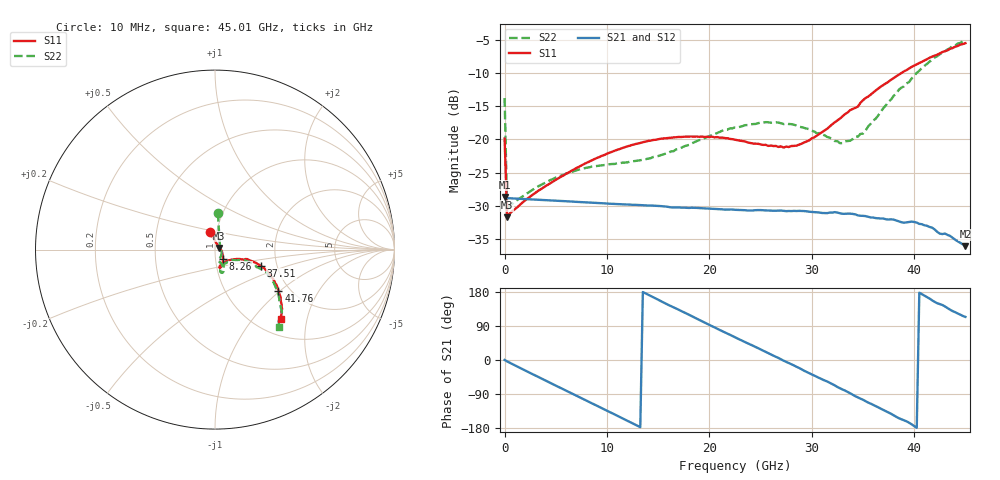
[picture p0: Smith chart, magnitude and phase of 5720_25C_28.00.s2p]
! Device:  ADRF5720
! Description: 0.5dB LSB GaAs MMIC 6-bit Digital Attenuator
! Frequency:  0.000009 -  40 GHz
! Ports:
!	RF1	= Port 1
!	RF2	= Port 2
! Vdd:  3.3 Volt
! Vss:  -3.3 Volt
! Control:  0/3.3 Volt
! State:  28.00 dB attenuation
! Data:  The device was measured using G-S-G Probes on a matrix board.
!  Data was collected using an calibrated 4 port network analyzer.
!  The reference plane for this measurement is at the launchers.
! Note:  Analog Devices supplies this data as a sample of measured data
!  for this product.  Your particular data for this product may vary.
!  Data was taken at 25 degrees C.
!  Analog Devices reserves the right to change this data at anytime.
# GHZ S DB R 45.0
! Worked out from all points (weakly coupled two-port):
!   181 points, 10 MHz to 45.01 GHz, reference 45 ohm
!   highest |S21| = -28.67 dB at 10 MHz (marker M1); lowest = -36.1 dB at 45.01 GHz (marker M2)
!   lowest |S11| = -31.7 dB at 260 MHz (marker M3), VSWR 1.05, Z = 47.2 + j0.883 ohm
!   |S11| at or under -10 dB: start of sweep to 38.75 GHz
!   |S22| runs from -30.6 to -5.1 dB; largest |S21 - S12| = 0.0001
!   S11 on the Smith chart (normalised r, x): 10 MHz: 0.93, +0.18; 8.26 GHz: 1.09, -0.11; 37.51 GHz: 1.65, -0.33; 41.76 GHz: 1.75, -0.97; 45.01 GHz: 1.30, -1.40
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0.01  -19.88 106.9  -28.67 0.1  -28.66 0.1  -13.78 85.6
0.26  -31.71 21.1  -28.85 -3.7  -28.85 -3.7  -30.62 15.6
3.26  -27.78 -17.5  -29.08 -44.3  -29.08 -44.3  -27.10 -35.2
7.76  -23.72 -46.2  -29.47 -104.0  -29.47 -104.0  -24.36 -68.5
8.26  -23.35 -48.5  -29.52 -110.6  -29.51 -110.6  -24.21 -70.0
12.01  -21.04 -62.0  -29.81 -160.4  -29.81 -160.4  -23.45 -74.4
15.26  -19.90 -69.9  -30.05 155.5  -30.05 155.5  -22.37 -68.8
20.26  -19.58 -75.8  -30.46 89.2  -30.46 89.2  -19.35 -63.6
22.76  -20.13 -75.0  -30.63 56.7  -30.63 56.8  -18.18 -66.4
25.51  -20.82 -65.5  -30.70 21.2  -30.70 21.2  -17.40 -71.8
27.26  -21.23 -56.3  -30.76 -1.8  -30.76 -1.8  -17.69 -74.3
30.26  -19.68 -33.4  -30.96 -41.0  -30.96 -41.0  -18.81 -74.5
32.76  -16.87 -21.4  -31.13 -74.6  -31.14 -74.6  -20.57 -60.0
33.76  -15.59 -19.5  -31.19 -87.8  -31.19 -87.8  -20.20 -46.3
34.51  -15.06 -17.3  -31.45 -98.8  -31.45 -98.7  -19.58 -38.7
35.01  -14.10 -17.0  -31.52 -104.9  -31.52 -104.9  -19.13 -33.2
37.51  -11.30 -19.7  -32.07 -138.5  -32.07 -138.5  -14.32 -19.9
37.76  -11.00 -20.3  -32.04 -142.1  -32.01 -142.1  -13.97 -19.5
40.26  -8.69 -27.4  -32.53 -178.8  -32.53 -178.7  -9.98 -23.8
41.76  -7.52 -32.8  -33.30 157.5  -33.30 157.4  -8.02 -31.8
43.76  -6.24 -40.5  -34.84 129.1  -34.82 129.3  -5.84 -43.1
45.01  -5.50 -46.5  -36.09 113.8  -36.07 113.7  -5.09 -50.4
